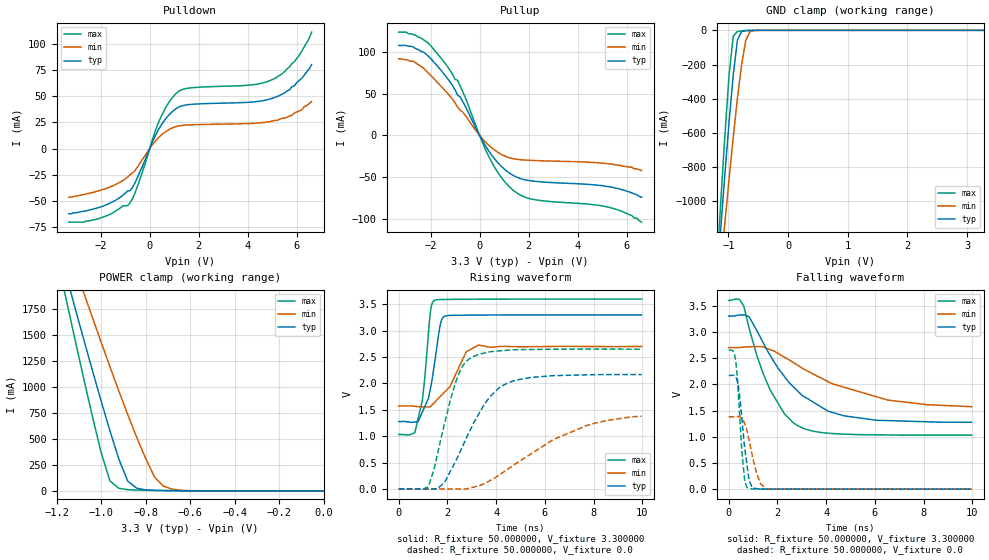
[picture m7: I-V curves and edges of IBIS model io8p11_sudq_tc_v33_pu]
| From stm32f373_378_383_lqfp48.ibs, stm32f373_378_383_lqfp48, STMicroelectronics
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|   Model io8p11_sudq_tc_v33_pu
[Model]  io8p11_sudq_tc_v33_pu
Model_type I/O
Polarity   Non-Inverting
Enable   Active-Low
Vinl =   0.990000V
Vinh =   2.310000V
Vmeas =  1.650000V
Cref =   30.000000pF
Rref =   100.000000M
Vref =   0.0V
C_comp   1.325200pF   1.251200pF   1.426700pF
[Temperature Range]   25.000000   0.125000k   -40.000000
[Pullup Reference]   3.300000V   2.700000V   3.600000V
[Pulldown Reference]   0.0V   0.0V   0.0V
[POWER Clamp Reference]   3.300000V   2.700000V   3.600000V
[GND Clamp Reference]   0.0V   0.0V   0.0V
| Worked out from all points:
|   slope of the pulldown table from 0 to 0.495 V, typ, clamps not added: 21.3 ohm
|   slope of the pullup table from 0 to 0.495 V, typ, clamps not added: 20.9 ohm
|   GND clamp passes 1 mA (typ) near -0.67 V on its own axis
|   POWER clamp passes 1 mA (typ) near -0.60 V on its own axis
|   rising waveform, R_fixture 50.000000, V_fixture 3.300000: 20-80 % time 440ps typ, 838ps min, 340ps max; typ from 1.28 V to 3.3 V
|   rising waveform, R_fixture 50.000000, V_fixture 0.0: 20-80 % time 1.49ns typ, 3.04ns min, 882ps max; typ from 0.001 V to 2.17 V
|   falling waveform, R_fixture 50.000000, V_fixture 3.300000: 20-80 % time 2.09ns typ, 3.36ns min, 1.32ns max; typ from 3.3 V to 1.28 V
|   falling waveform, R_fixture 50.000000, V_fixture 0.0: 20-80 % time 301ps typ, 417ps min, 225ps max; typ from 2.17 V to 0.001 V
[Pulldown]
|Voltage   I(typ)   I(min)   I(max)
-3.3V     -62mA      -46.3mA    -70mA
-2.1V     -56.2mA    -40.3mA    -66.8mA
-800mV    -40.05mA   -24.9mA    -51.58mA
-500mV    -27.57mA   -17.6mA    -36.07mA
400mV     19.71mA    11.36mA    27.01mA
700mV     29.83mA    16.93mA    40.97mA
1.1V      38.46mA    21.2mA     53.02mA
1.6V      41.98mA    22.62mA    57.7mA
4.1V      44.26mA    24mA       60.59mA
5V        48mA       26.2mA     65.8mA
5.9V      60mA       34mA       83mA
6.6V      80mA       45mA       111mA
[Pullup]
|Voltage   I(typ)   I(min)   I(max)
-3.3V     108mA      92mA       124mA
-2.7V     106mA      89mA       121mA
-2.2V     98mA       78.1mA     113mA
-1.4V     71.8mA     53.5mA     86.1mA
-900mV    48.5mA     34.23mA    66.14mA
-700mV    41.33mA    28.36mA    53.31mA
400mV     -19.77mA   -12.52mA   -26.8mA
900mV     -37.48mA   -22.89mA   -50.99mA
1.4V      -48.39mA   -28.06mA   -66.43mA
2.2V      -54.79mA   -29.98mA   -76.75mA
5.3V      -61.6mA    -34.1mA    -86.4mA
6.6V      -74mA      -42mA      -104mA
[GND_clamp]
|Voltage   I(typ)   I(min)   I(max)
-3.3V     -9.739A    -9.975A    -9.587A
-1.2V     -1.489A    -1.65A     -1.416A
-1.13V    -1.162A    -1.385A    -1.009A
-1.06V    -842.2mA   -1.125A    -616.9mA
-990mV    -537.1mA   -870.1mA   -263mA
-920mV    -262.4mA   -625.3mA   -33.96mA
-850mV    -56.94mA   -397.4mA   -7.08mA
-780mV    -7.011mA   -202.2mA   -3.71mA
-710mV    -1.778mA   -58.23mA   -1.736mA
-640mV    -550uA     -8.783mA   -542.4uA
-570mV    -109.8uA   -1.292mA   -86.89uA
3.28V     0A         0A         0A
[POWER_clamp]
|Voltage   I(typ)   I(min)   I(max)
-3.28V    9.897A     9.838A     9.594A
-1.16V    2.103A     2.419A     1.88A
-1.12V    1.788A     2.17A      1.488A
-1.08V    1.476A     1.923A     1.102A
-1V       868.2mA    1.435A     373.1mA
-960mV    578.3mA    1.196A     96.08mA
-880mV    93.25mA    734.2mA    12.03mA
-840mV    26.31mA    517.4mA    8.576mA
-760mV    5.12mA     134mA      5.134mA
-720mV    3.368mA    46.35mA    3.823mA
-600mV    1.018mA    2.575mA    1.086mA
0V        0A         0A         0A
[Ramp]
| variable   typ   min   max
dV/dt_r  1.30001/1.48830n   0.78791/3.04596n   1.58840/0.88090n
dV/dt_f  1.21410/2.09201n   0.66018/3.37829n   1.54158/1.31557n
R_load = 50.000000
[Rising Waveform]
R_fixture= 50.000000
V_fixture= 3.300000
V_fixture_min= 2.700000
V_fixture_max= 3.600000
|time   V(typ)   V(min)   V(max)
0s        1.277V     1.573V     1.031V
660.7ps   1.269V     1.566V     1.065V
981ps     1.465V     1.555V     1.71V
1.301ns   1.898V     1.56V      3.351V
1.461ns   2.352V     1.636V     3.574V
1.742ns   3.179V     1.768V     3.591V
1.942ns   3.282V     1.862V     3.593V
2.763ns   3.294V     2.592V     3.596V
3.263ns   3.296V     2.724V     3.598V
9.97ns    3.3V       2.7V       3.6V
[Rising Waveform]
R_fixture= 50.000000
V_fixture= 0.0
V_fixture_min= 0.0
V_fixture_max= 0.0
|time   V(typ)   V(min)   V(max)
0s        1mV        1.1mV      956.6uV
1.221ns   -3.482mV   932.5uV    44.6mV
1.461ns   -717.6uV   176uV      386.9mV
1.882ns   120.9mV    -1.493mV   1.234V
2.402ns   584.6mV    -1.707mV   2.106V
3.043ns   1.217V     29.57mV    2.505V
3.744ns   1.745V     156.5mV    2.601V
4.725ns   2.048V     453mV      2.639V
7.728ns   2.163V     1.203V     2.65V
9.97ns    2.168V     1.379V     2.649V
[Falling Waveform]
R_fixture= 50.000000
V_fixture= 3.300000
V_fixture_min= 2.700000
V_fixture_max= 3.600000
|time   V(typ)   V(min)   V(max)
0s        3.3V       2.7V       3.6V
600.6ps   3.324V     2.707V     3.508V
840.8ps   3.285V     2.716V     3.069V
1.161ns   3.018V     2.719V     2.542V
1.702ns   2.549V     2.66V      1.893V
2.282ns   2.152V     2.519V     1.441V
2.803ns   1.885V     2.371V     1.22V
4.745ns   1.398V     1.942V     1.05V
6.547ns   1.308V     1.698V     1.034V
9.97ns    1.277V     1.573V     1.031V
[Falling Waveform]
R_fixture= 50.000000
V_fixture= 0.0
V_fixture_min= 0.0
V_fixture_max= 0.0
|time   V(typ)   V(min)   V(max)
0s        2.168V     1.379V     2.649V
280.3ps   2.146V     1.383V     2.471V
400.4ps   1.956V     1.385V     1.787V
560.6ps   1.26V      1.342V     616.9mV
660.7ps   779.4mV    1.243V     160.1mV
800.8ps   290.8mV    1.013V     17.18mV
961ps     33.97mV    663.9mV    5.863mV
1.121ns   12.33mV    344.5mV    3.814mV
1.562ns   3.858mV    7.281mV    2.527mV
9.97ns    1mV        1.1mV      956.6uV
